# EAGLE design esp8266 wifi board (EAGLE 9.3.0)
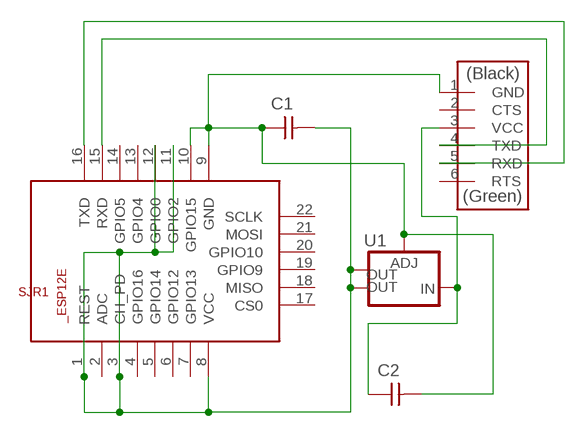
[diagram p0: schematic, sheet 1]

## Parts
C1  CAP-UNPOLARIZEDFAB  [C1206FAB]
C2  CAP-UNPOLARIZEDFAB  [C1206FAB]
SJR1  ESP8266-12EESP12E  [ESP8266-ESP12E]
U1  V_REG_LM1117SOT223  [SOT223]
U$1  FTDI-SMD-HEADER  [1X06SMD]

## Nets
N$1: C1.1 C2.2 SJR1.9(GND) SJR1.10(GPIO15) U1.1(ADJ) U$1.1(GND)
N$2: C2.1 U1.3(IN) U$1.3(VCC)
N$5: SJR1.16(TXD) U$1.5(RXD)
N$6: SJR1.15(RXD) U$1.4(TXD)
N$7: C1.2 SJR1.1(REST) SJR1.3(CH_PD) SJR1.8(VCC) SJR1.11(GPIO2) SJR1.12(GPIO0) U1.2(OUT) U1.4(OUT)
Unconnected: SJR1.2(ADC) SJR1.4(GPIO16) SJR1.5(GPIO14) SJR1.6(GPIO12) SJR1.7(GPIO13) SJR1.13(GPIO4) SJR1.14(GPIO5) SJR1.17(CS0) SJR1.18(MISO) SJR1.19(GPIO9) SJR1.20(GPIO10) SJR1.21(MOSI) SJR1.22(SCLK) U$1.2(CTS) U$1.6(RTS)

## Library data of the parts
C1 C2 = fab:CAP-UNPOLARIZED
SJR1 = esp12e:ESP8266-12E: ESP8266-12E Library for Eagle CAD The author not responsible for any damages or errors!. Created by Suhail jr.lt;/author>
U1 = fab:V_REG_LM1117: Voltage Regulator LM1117 Standard adjustable voltage regulator but in SMD form. Spark Fun Electronics SKU : COM-00595; PROD_ID: VREG-08170
U$1 = fab:FTDI-SMD-HEADER

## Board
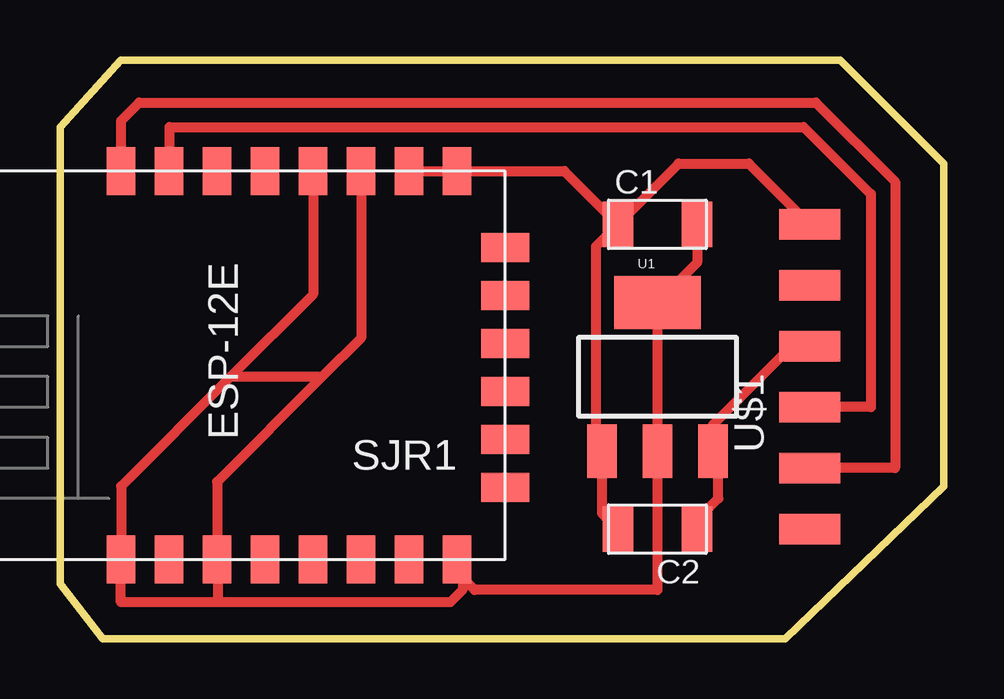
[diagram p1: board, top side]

Size 36.83 x 24.13 mm. Coordinates in mm from the lower left corner, seen from the top.
Outline: 2.54,24.13 32.51,24.13 36.83,19.81 36.83,6.35 30.23,0 1.78,0 0,2.29 0,21.34 2.54,24.13
Copper layers (1*16): Top 0.035mm / dielectric 1.5mm / Bottom 0.035mm
Design rules "fabmodule": minimum track width 10mil, minimum drill 0.4mm, track to track 0.42mm, track to pad 0.42mm, pad to pad 0.42mm, via to via 0.42mm, smd to smd 0.42mm, copper to edge 40mil, drill to drill 0.8mm, minimum pad ring 10mil, minimum via ring 8mil, stop-mask expansion 4mil, vias tented up to drill 0mil, thermal gap 10mil

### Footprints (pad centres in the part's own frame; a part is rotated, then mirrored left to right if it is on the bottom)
C1206FAB = smd 1.27 x 1.905: 1 -1.651,0; 2 1.651,0
ESP8266-ESP12E = smd 2 x 1.2: 1 -7.62,5.84; 2 -7.62,3.84; 3 -7.62,1.84; 4 -7.62,-0.16; 5 -7.62,-2.16; 6 -7.62,-4.16; 7 -7.62,-6.16; 8 -7.62,-8.16; 9 8.58,-8.16; 10 8.58,-6.16; 11 8.58,-4.16; 12 8.58,-2.16; 13 8.58,-0.16; 14 8.58,1.84; 15 8.58,3.84; 16 8.58,5.84 | smd 1.2 x 2: 17 -4.62,-10.16; 18 -2.62,-10.16; 19 -0.62,-10.16; 20 1.38,-10.16; 21 3.38,-10.16; 22 5.38,-10.16
SOT223 = smd 1.219 x 2.235: 1 -2.311,-3.099; 2 0,-3.099; 3 2.311,-3.099 | smd 3.6 x 2.2: 4 0,3.099
1X06SMD = smd 2.54 x 1.27: 1 0,6.35; 2 0,3.81; 3 0,1.27; 4 0,-1.27; 5 0,-3.81; 6 0,-6.35

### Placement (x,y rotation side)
C1  24.89,17.27 0 top
C2  24.89,4.57 180 top
SJR1  8.38,10.92 90 top
U1  24.89,10.92 0 top
U$1  31.24,10.92 0 top

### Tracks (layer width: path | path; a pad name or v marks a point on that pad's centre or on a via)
N$1
  Top 0.406: C1.1 21.01,19.5 SJR1.9 SJR1.10 | C1.1 25.78,19.81 28.7,19.81 U$1.1 | C1.1 22.33,16.36 22.33,8.08 U1.1 22.58,5.23 C2.2
N$2
  Top 0.406: C2.1 26.54,4.95 27.43,5.84 27.43,7.59 U1.3 27.2,8.91 30.73,12.45 30.99,12.19 U$1.3
N$5
  Top 0.406: SJR1.16 2.54,21.59 3.3,22.35 31.5,22.35 34.8,19.05 34.8,7.11 U$1.5
N$6
  Top 0.406: SJR1.15 4.57,19.53 4.57,21.34 30.99,21.34 33.78,18.54 33.78,9.65 U$1.4
N$7
  Top 0.406: C1.2 26.54,15.67 U1.4 U1.2 24.89,2.03 17.27,2.03 16.54,2.76 SJR1.8 16.78,3.06 16.78,2.04 16.26,1.52 6.6,1.52 | SJR1.11 12.54,12.54 10.92,10.92 | 10.92,10.92 6.54,6.54 SJR1.3 6.6,3.24 6.6,1.52 | SJR1.12 10.54,14.35 7.11,10.92 | 7.11,10.92 2.54,6.35 SJR1.1 2.54,1.52 6.6,1.52 | 7.11,10.92 10.92,10.92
